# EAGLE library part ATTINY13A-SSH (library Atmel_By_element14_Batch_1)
8-bit Microcontroller with In-System Programmable Flash
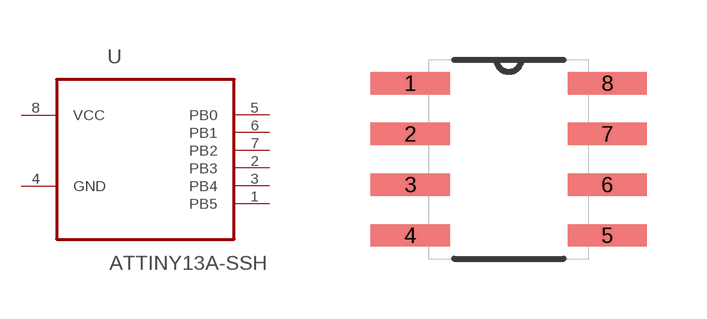
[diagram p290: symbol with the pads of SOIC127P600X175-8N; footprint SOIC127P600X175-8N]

Designator prefix U

## ATTINY13A-SSH (MPN: ATTINY13A-SSH; OC_FARNELL: 1715519; OC_NEWARK: 15R0301; PACKAGE: SOIC-8; SUPPLIER: Atmel)  [SOIC127P600X175-8N]
1  PB5
2  PB3
3  PB4
4  GND  pas
5  PB0
6  PB1
7  PB2
8  VCC  pwr

## Footprint SOIC127P600X175-8N (pad centres in mm)
smd 1.981 x 0.559: 1 -2.464,1.905; 2 -2.464,0.635; 3 -2.464,-0.635; 4 -2.464,-1.905; 5 2.464,-1.905; 6 2.464,-0.635; 7 2.464,0.635; 8 2.464,1.905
